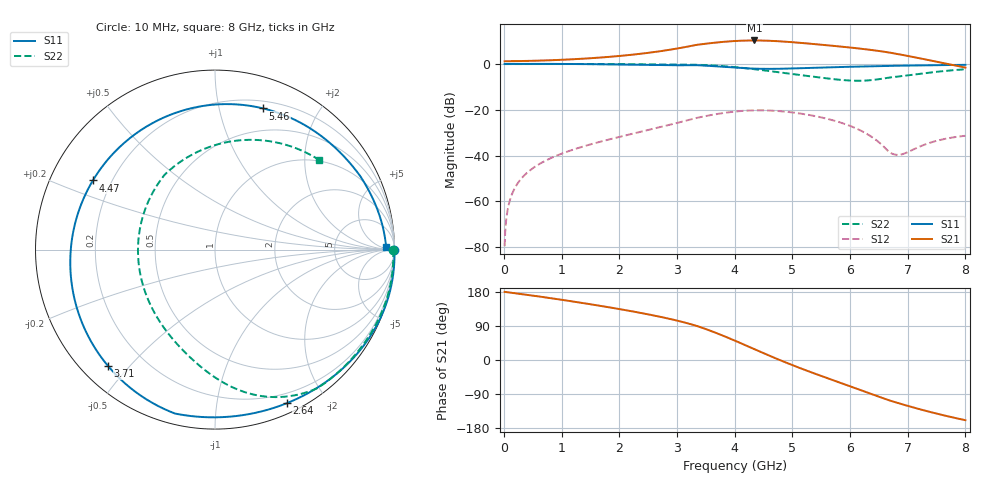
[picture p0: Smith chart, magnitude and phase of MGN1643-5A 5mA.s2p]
! Port[1] = GATE
! Port[2] = DRAIN
! [Type]  S-parameter s2p file touchstone ver. 1.0
! [Object]  MGN1643-5A
! [Bias]  5 mA
! [Version]  1.0
! [Date]  Thu May 19 11:02:03 2026
! [Source]  This file was created in JSC "ICC Milandr".
! [Disclaimer] Property of JSC "ICC Milandr". Unauthorized reproduction and/or distribution is strictly prohibited.
!  The file and the data are provided "AS IS" and with all faults and disclaim all warranties, express and implied, including
!  without limitation any implied warranties of merchantability, fitness for a particular purpose.
!  JSC "ICC Milandr" assumes no liability for:
!  1) the accuracy of the data provided;
!  2) the proper functioning of this data;
!  3) infringement of patents, copyrights or intellectual property rights resulting from the use of this data.
!  JSC "ICC Milandr" reserves the right to make changes to the products and the data without prior notice.
!  Please, be aware that your receipt and use of the file provided shall serve as acceptance of these terms and conditions.
!  If you do not accept these terms, you should return or destroy this file and any other accompanying information immediately.
# Hz S MA R 12.5
! freq  S11mag  S11ang  S21mag  S21ang  S12mag  S12ang  S22mag  S22ang
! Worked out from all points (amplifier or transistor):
!   800 points, 10 MHz to 8 GHz, reference 12.5 ohm
!   highest |S21| = 10.2 dB at 4.34 GHz (marker M1)
!   |S21| within 3 dB of that: 3.117 GHz to 5.969 GHz (2.851 GHz wide, 62.8 % of centre)
!   unconditionally stable (mu >= 1): 6.107 GHz to 7.743 GHz
!   at 1.34 GHz: K = 0.16, MSG = 19.3 dB, |S12| = -36.3 dB
!   at 4.01 GHz: K = 0.41, MSG = 15.4 dB, |S12| = -20.8 dB
!   at 8 GHz: K = 0.81, MSG = 14.9 dB, |S12| = -31.3 dB
!   S11 on the Smith chart (normalised r, x): 10 MHz: open; 2.64 GHz: 0.10, -1.57; 3.71 GHz: 0.08, -0.44; 4.47 GHz: 0.13, +0.26; 5.46 GHz: 0.27, +1.36; 8 GHz: 39, +11
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1e7  1 -0.2  1.147 179.8  0.0001054 87.0  0.9928 -0.1
1.1e8  1.001 -2.1  1.149 177.9  0.001151 87.9  0.9936 -1.4
3.1e8  1.002 -5.8  1.157 173.8  0.003259 84.8  0.995 -3.9
7e8  1.002 -13.4  1.189 165.6  0.007517 78.2  0.9965 -8.9
1.35e9  0.9932 -27.0  1.296 150.7  0.01548 66.0  0.9944 -17.6
2.64e9  0.9448 -64.9  1.842 116.2  0.03981 36.1  0.9755 -37.9
2.68e9  0.9433 -66.5  1.872 114.9  0.04094 35.0  0.9747 -38.7
3.25e9  0.9365 -97.2  2.477 94.0  0.06201 15.4  0.9622 -51.3
3.47e9  0.921 -113.0  2.735 83.2  0.07172 5.2  0.9449 -57.2
3.71e9  0.8808 -132.5  2.955 69.5  0.08137 -7.3  0.9102 -64.1
4.01e9  0.8292 -161.0  3.166 50.6  0.09144 -24.2  0.8504 -73.2
4.34e9  0.789 164.2  3.252 28.7  0.09702 -43.6  0.7679 -83.4
4.47e9  0.7819 150.5  3.238 20.0  0.09718 -51.1  0.7335 -87.4
4.85e9  0.7875 113.9  3.075 -4.4  0.09152 -71.7  0.6368 -99.8
5.34e9  0.8222 78.0  2.741 -33.2  0.07487 -94.5  0.5305 -120.3
5.46e9  0.8311 71.1  2.656 -39.9  0.06983 -99.5  0.5077 -126.8
5.75e9  0.8511 56.9  2.453 -55.7  0.05664 -110.7  0.4599 -146.1
6.04e9  0.869 45.4  2.253 -71.5  0.04243 -120.8  0.4315 -171.2
6.67e9  0.9073 26.7  1.782 -106.1  0.01203 -123.8  0.5029 123.8
6.87e9  0.9153 22.3  1.605 -115.3  0.01045 -93.2  0.5376 106.3
7.23e9  0.93 14.9  1.312 -130.8  0.01612 -65.1  0.6149 79.9
8e9  0.9541 0.7  0.8319 -158.9  0.02707 -71.6  0.7652 40.8
